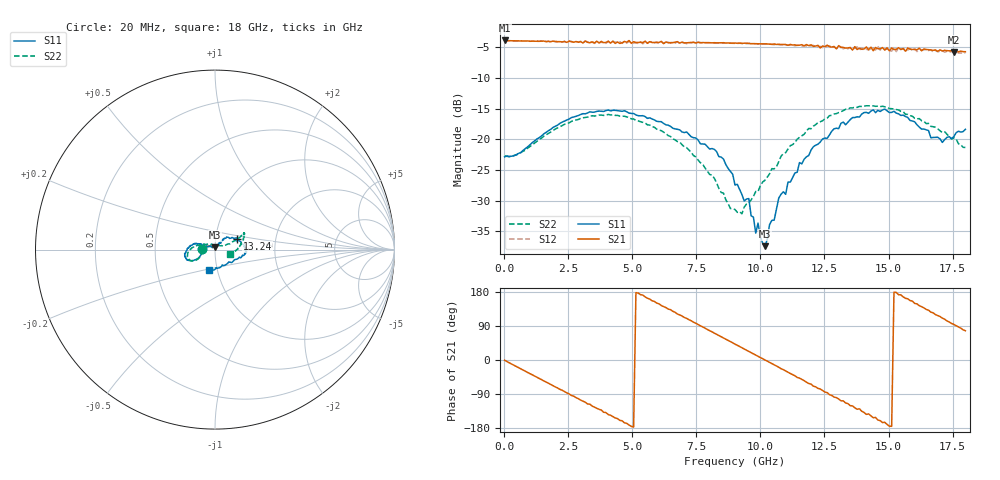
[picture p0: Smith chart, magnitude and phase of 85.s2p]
!Agilent Technologies,N5230A,US43500223,A.07.50.48
!Agilent N5230A: A.07.50.48
!Date: Thursday, January 14, 2016 16:38:00
!Correction: S11(Full 2 Port(1,2))
!S21(Full 2 Port(1,2))
!S12(Full 2 Port(1,2))
!S22(Full 2 Port(1,2))
!S2P File: Measurements: S11, S21, S12, S22:
# Hz S  dB  R 50
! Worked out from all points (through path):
!   201 points, 20 MHz to 18 GHz, reference 50 ohm
!   highest |S21| = -3.91 dB at 20 MHz (marker M1); lowest = -5.8 dB at 17.55 GHz (marker M2)
!   group delay of S21, straight-line fit = 98.9 ps
!   lowest |S11| = -37.4 dB at 10.18 GHz (marker M3), VSWR 1.03, Z = 49.8 + j1.34 ohm
!   |S11| at or under -10 dB: start of sweep to end of sweep
!   |S22| runs from -32.1 to -14.5 dB; largest |S21 - S12| = 0.061
!   S11 on the Smith chart (normalised r, x): 20 MHz: 0.87, +0.00; 13.24 GHz: 1.28, +0.15; 18 GHz: 0.91, -0.21
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2e7  -22.86 179.5  -3.91 -0.8  -3.93 -0.9  -22.67 179.4
1.7281e9  -18.60 -152.6  -4.07 -61.2  -4.03 -62.0  -19.04 -150.8
3.0766e9  -15.83 -158.7  -4.32 -108.6  -4.26 -109.4  -16.50 -155.6
4.515e9  -15.39 -170.7  -4.40 -159.4  -4.12 -160.9  -16.22 -170.2
4.8746e9  -15.73 -174.2  -3.93 -171.6  -4.04 -171.5  -16.45 -174.3
6.0433e9  -17.12 172.0  -4.23 148.3  -4.44 146.7  -18.48 172.4
7.5716e9  -20.13 160.4  -4.21 93.5  -4.19 92.7  -23.39 152.3
8.5605e9  -23.21 161.5  -4.28 58.1  -4.34 56.5  -28.75 121.5
9.01e9  -27.43 160.0  -4.34 41.8  -4.37 40.1  -31.43 86.9
9.5494e9  -29.64 143.2  -4.38 22.7  -4.40 20.7  -30.37 54.7
9.8191e9  -35.26 143.2  -4.45 12.9  -4.45 10.8  -28.49 35.7
9.909e9  -33.63 121.1  -4.45 9.8  -4.49 7.5  -28.52 33.9
1.01787e10  -37.39 95.7  -4.46 0.1  -4.53 -2.1  -26.66 26.7
1.07181e10  -29.55 59.1  -4.53 -19.1  -4.60 -21.6  -23.63 22.7
1.20666e10  -21.21 46.4  -4.87 -68.9  -4.73 -70.0  -17.86 25.8
1.32353e10  -17.20 25.2  -5.04 -107.8  -5.27 -112.2  -15.33 28.1
1.41343e10  -15.62 5.1  -4.97 -143.5  -5.32 -143.2  -14.54 29.4
1.50333e10  -15.64 -6.2  -5.61 -174.6  -5.54 -177.4  -14.99 26.1
1.6202e10  -18.02 -25.9  -5.18 143.4  -5.46 142.1  -16.64 10.5
1.7101e10  -20.50 -65.2  -5.62 110.4  -5.61 106.1  -18.89 -2.8
1.75505e10  -19.55 -86.7  -5.80 93.8  -5.96 89.4  -19.75 -7.6
1.8e10  -18.38 -106.5  -5.75 77.2  -5.95 72.9  -21.33 -14.7
